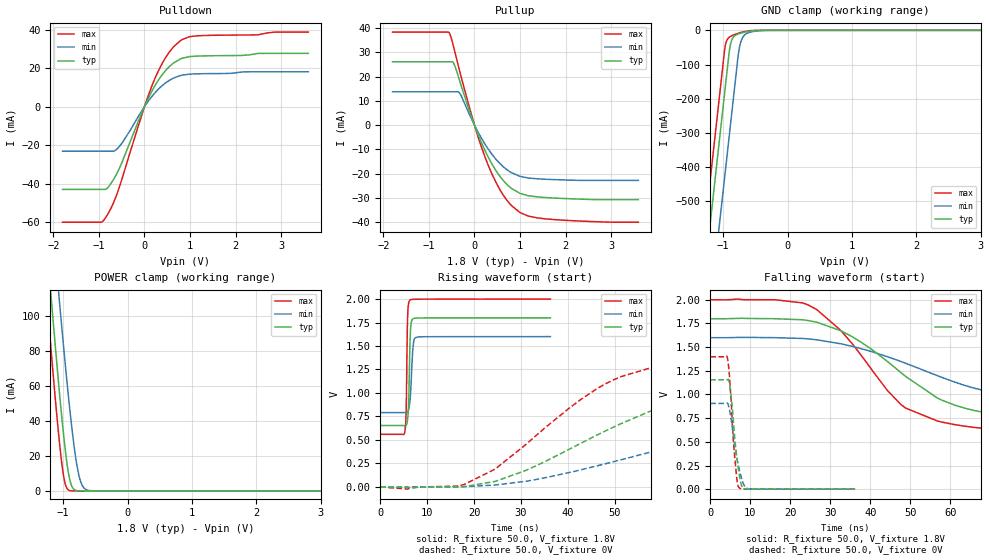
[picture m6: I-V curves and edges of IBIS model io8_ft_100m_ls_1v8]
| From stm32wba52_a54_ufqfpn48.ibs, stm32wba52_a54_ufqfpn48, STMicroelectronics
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[Model]   io8_ft_100m_ls_1v8
Model_type I/O
Polarity   Non-Inverting
Enable   Active-Low
| CAP_THRESHOLD on pad IOFT is "UDTCAPC" :
| Rising=30.0% of vddiom   Falling=70.0% of vddiom
| C_comp min and max val. don't necessarily correlate with the min and max pvt
| but are the smallest and greatest pad capacitance found.
| var   typ   min   max
C_comp   2.20762pF  2.09928pF  2.39593pF
|C_comp_pullup   1.38155pF  1.31740pF  1.46386pF
|C_comp_pulldown   826.06519fF  781.87502fF  932.07109fF
Vinl = 800.0mV
Vinh = 1.0V
Vmeas = 900.0mV   | Reference voltage for timing measurements
Cref  = 50.0pF   | Timing specification test load capacitance value
Rref  = 1.0MOhm   | Timing specification test load resistance value
Vref  = 990.0mV   | Timing specification test load voltage
[Model Spec]
| TIME_THRESHOLD on pin ZIV11 is "CMOS" :
| Rising=50.0% of vdd   Falling=50.0% of vdd
Vinl 702.50000mV 642.50000mV 771.50000mV
Vinh 1.09050V 944.50000mV 1.21950V
| variable   typ   min   max
[Temperature Range] 25.0 140.0 -40.0
| variable   typ   min   max
[Voltage Range] 1.8V 1.6V 2.0V
| variable   typ   min   max
[POWER Clamp Reference] 1.8V 1.6V 2.0V
| variable   typ   min   max
[GND Clamp Reference] 0V 0V 0V
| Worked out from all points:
|   slope of the pulldown table from 0 to 0.27 V, typ, clamps not added: 21.7 ohm
|   slope of the pullup table from 0 to 0.27 V, typ, clamps not added: 22.5 ohm
|   GND clamp passes 1 mA (typ) near -0.51 V on its own axis
|   POWER clamp passes 1 mA (typ) near -0.83 V on its own axis
|   rising waveform, R_fixture 50.0, V_fixture 1.8V: 20-80 % time 320ps typ, 504ps min, 248ps max; typ from 0.654 V to 1.8 V
|   falling waveform, R_fixture 50.0, V_fixture 1.8V: 20-80 % time 24.5ns typ, 38.3ns min, 17.7ns max; typ from 1.8 V to 0.654 V
|   rising waveform, R_fixture 50.0, V_fixture 0V: 20-80 % time 31.2ns typ, 49.2ns min, 22.1ns max; typ from 0 V to 1.16 V
|   falling waveform, R_fixture 50.0, V_fixture 0V: 20-80 % time 1.6ns typ, 2.13ns min, 1.33ns max; typ from 1.16 V to 0 V
[POWER Clamp]
-1.8V     396.4mA    438.1mA    365.5mA
-1.26V    143.5mA    194.6mA    112.6mA
-1.19V    112.3mA    164.2mA    81.56mA
-1.06V    57.23mA    109.3mA    28.68mA
-1.02V    41.75mA    93.06mA    15.5mA
-980mV    27.6mA     77.28mA    5.935mA
-910mV    8.693mA    51.24mA    382.3uA
-850mV    1.642mA    31.41mA    23.97uA
-760mV    69.41uA    9.714mA    358.6nA
-700mV    7.83uA     2.919mA    21.79nA
-620mV    424.6nA    410.3uA    573.9pA
3.6V      0A         0A         0A
[GND Clamp]
-1.8V     -1.583A    -1.83A     -1.456A
-1.43V    -953.9mA   -1.201A    -826.8mA
-1.24V    -630.9mA   -877.8mA   -503.8mA
-1.05V    -307.9mA   -554.8mA   -180.8mA
-970mV    -171.9mA   -418.8mA   -48.31mA
-910mV    -69.87mA   -316.8mA   -20.91mA
-880mV    -36.5mA    -265.8mA   -17.19mA
-830mV    -17.68mA   -180.8mA   -12.97mA
-750mV    -9.66mA    -53.66mA   -7.697mA
-690mV    -6.479mA   -19.19mA   -4.622mA
-600mV    -3.058mA   -6.478mA   -1.59mA
3.6V      1.281nA    1.39uA     517.2pA
| variable   typ   min   max
[Pullup Reference] 1.8V 1.6V 2.0V
| variable   typ   min   max
[Pulldown Reference] 0V 0V 0V
[Pullup]
-1.8V     26.12mA    13.77mA    38.36mA
-560mV    26.12mA    13.77mA    38.22mA
-460mV    25.58mA    13.77mA    32.35mA
-330mV    18.52mA    13.29mA    22.64mA
20mV      -1.006mA   -751.6uA   -1.259mA
280mV     -12.36mA   -9.262mA   -15.51mA
450mV     -18.1mA    -13.58mA   -22.78mA
630mV     -22.78mA   -17.1mA    -28.78mA
810mV     -26.07mA   -19.57mA   -33.13mA
1V        -28.15mA   -21.12mA   -36.04mA
1.6V      -29.9mA    -22.35mA   -38.71mA
3.6V      -30.74mA   -22.8mA    -40.02mA
[Pulldown]
-1.8V     -42.97mA   -23.15mA   -59.99mA
-950mV    -42.97mA   -23.15mA   -59.99mA
-850mV    -42.87mA   -23.15mA   -57.45mA
-670mV    -37.41mA   -23.03mA   -49.3mA
-550mV    -31.91mA   -20.61mA   -41.6mA
10mV      539.8uA    356.7uA    722uA
230mV     10.88mA    7.174mA    14.64mA
500mV     19.69mA    12.93mA    26.79mA
790mV     24.78mA    16.15mA    34.26mA
1V        26.02mA    16.89mA    36.38mA
1.18V     26.27mA    17.05mA    36.82mA
3.6V      27.68mA    18.11mA    38.71mA
[Ramp]
dV/dt_r 693.10111mV/31.1293ns 543.32588mV/48.95035ns 838.83184mV/21.888ns
dV/dt_f 687.72957mV/24.37234ns 485.01762mV/38.23221ns 864.01404mV/17.33608ns
R_load = 50.0
| Removed startup time: 0s 0s 0s  .
| Removed end time: 36.25ns.
[Rising Waveform]
R_fixture   = 50.0
V_fixture   = 1.8V
V_fixture_min = 1.6V
V_fixture_max = 2.0V
0s        653.8mV    791.8mV    560mV
5.2ns     651.6mV    790.6mV    579.2mV
5.5ns     654.1mV    788.9mV    782.7mV
5.75ns    695.3mV    793.6mV    1.65V
5.85ns    732.5mV    800.2mV    1.843V
6.05ns    901.3mV    828.1mV    1.958V
6.35ns    1.562V     927mV      1.989V
7ns       1.79V      1.499V     1.997V
7.6ns     1.797V     1.591V     1.998V
36.25ns   1.8V       1.6V       2V
| Removed startup time: 0s 0s 0s  .
| Removed end time: 399.25ns.
[Falling Waveform]
R_fixture   = 50.0
V_fixture   = 1.8V
V_fixture_min = 1.6V
V_fixture_max = 2.0V
0s        1.8V       1.6V       2V
24.45ns   1.781V     1.587V     1.946V
35.7ns    1.606V     1.506V     1.526V
44.3ns    1.349V     1.399V     1.042V
48.9ns    1.189V     1.329V     855.5mV
57.8ns    942mV      1.182V     709.5mV
70.9ns    792mV      1.017V     630.2mV
96.85ns   699.2mV    882.4mV    580.4mV
141.4ns   663mV      816.1mV    563mV
399.3ns   653.8mV    791.6mV    560mV
| Removed startup time: 0s 0s 0s  .
| Removed end time: 399.2ns.
[Rising Waveform]
R_fixture   = 50.0
V_fixture   = 0V
V_fixture_min = 0V
V_fixture_max = 0V
0s        4.66nV     680.4nV    3.931nV
17.8ns    3.285mV    2.879mV    24.41mV
24.45ns   58.08mV    20.07mV    188.8mV
31ns      175.5mV    59.6mV     450.7mV
48.2ns    601.3mV    249.5mV    1.103V
57.05ns   796.1mV    363.7mV    1.259V
71ns      996.7mV    534.6mV    1.346V
102.3ns   1.124V     783.6mV    1.391V
141.2ns   1.15V      873.6mV    1.398V
399.2ns   1.155V     905.5mV    1.398V
| Removed startup time: 0s 0s 0s  .
| Removed end time: 36.25ns.
[Falling Waveform]
R_fixture   = 50.0
V_fixture   = 0V
V_fixture_min = 0V
V_fixture_max = 0V
0s        1.155V     905.4mV    1.398V
4.25ns    1.155V     910.2mV    1.393V
5.05ns    1.043V     783mV      1.035V
5.7ns     759.9mV    592.1mV    558.8mV
6.15ns    524.2mV    452.8mV    321.6mV
6.7ns     312.4mV    313.8mV    90.67mV
7.15ns    177.3mV    225.6mV    16.95mV
8ns       20.15mV    88.95mV    3.079mV
9.65ns    1.67mV     3.028mV    1.007mV
36.25ns   215.3uV    205.3uV    176.7uV
